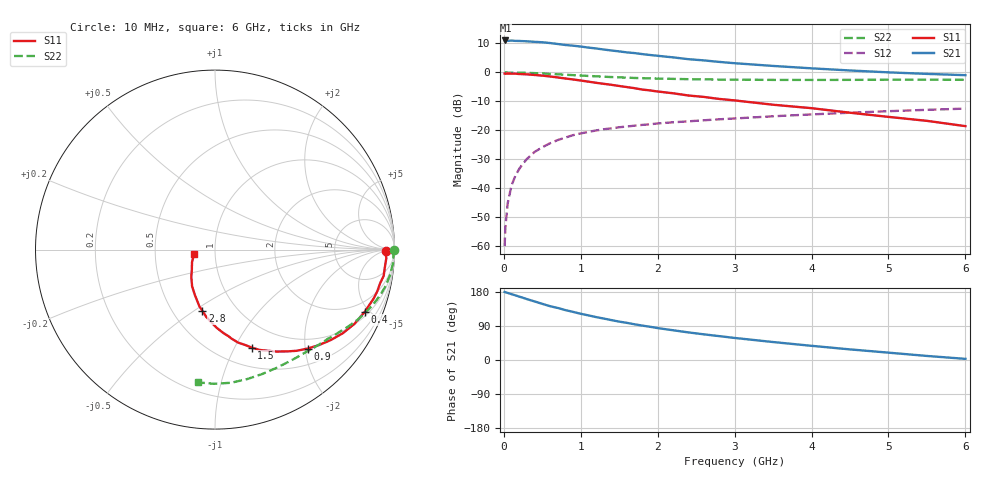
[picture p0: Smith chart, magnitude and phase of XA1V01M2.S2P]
! SIEMENS Discrete & RF Semiconductors
! BFY180
! Si NPN RF Bipolar Junction Transistor in MICRO-X
! VCE = 1 V  IC = 1.2 mA
! Common Emitter S-Parameters:  May  1997
# GHz  S  MA  R  50
!  f  S11  S21  S12  S22
! GHz  MAG  ANG  MAG  ANG  MAG  ANG  MAG  ANG
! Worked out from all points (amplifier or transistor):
!   36 points, 10 MHz to 6 GHz, reference 50 ohm
!   highest |S21| = 11.0 dB at 20 MHz (marker M1)
!   |S21| within 3 dB of that: start of sweep to 1.264 GHz
!   unconditionally stable (mu >= 1): 2.75 GHz to end of sweep
!   at 250 MHz: K = 0.10, MSG = 21.1 dB, |S12| = -31.5 dB
!   at 1.4 GHz: K = 0.65, MSG = 13.4 dB, |S12| = -19.3 dB
!   at 6 GHz: K = 1.12, MAG = 3.6 dB, |S12| = -12.5 dB
!   S11 on the Smith chart (normalised r, x): 10 MHz: 42, -8; 400 MHz: 1.24, -4.69; 900 MHz: 0.80, -2.05; 1.5 GHz: 0.71, -1.17; 2.8 GHz: 0.70, -0.54; 6 GHz: 0.79, -0.04
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0.01  0.955 -0.5  3.527 179.6  0.001 92.1  0.9953 -0.2
0.02  0.9488 -1.2  3.562 178.7  0.0021 86.0  0.9999 -0.6
0.05  0.9558 -2.8  3.506 177.0  0.0055 86.8  0.9951 -1.5
0.1  0.9515 -5.9  3.545 173.7  0.0112 86.2  0.9944 -3.1
0.2  0.9389 -11.5  3.491 167.2  0.0216 82.8  0.9895 -6.1
0.4  0.9032 -22.6  3.372 154.5  0.0424 74.8  0.9723 -12.0
0.5  0.8799 -28.1  3.316 148.2  0.051 71.0  0.9582 -14.7
0.6  0.851 -33.2  3.215 142.0  0.0597 67.9  0.9434 -17.3
0.9  0.7559 -46.8  2.894 127.0  0.0826 58.8  0.8978 -24.3
1  0.7245 -51.1  2.795 122.0  0.0885 56.5  0.884 -26.4
1.1  0.6927 -55.0  2.683 117.7  0.0939 54.3  0.8688 -28.3
1.2  0.6619 -59.1  2.589 113.2  0.0996 52.0  0.856 -30.2
1.5  0.5825 -69.5  2.305 101.3  0.113 46.9  0.821 -35.2
1.8  0.5053 -79.4  2.071 90.8  0.1242 43.2  0.7959 -39.7
2  0.4682 -84.1  1.936 84.2  0.1314 40.8  0.7833 -42.7
2.2  0.4365 -88.7  1.818 78.5  0.1377 38.5  0.7735 -45.6
2.6  0.3773 -97.5  1.612 67.7  0.1491 35.1  0.7573 -50.9
2.8  0.3484 -101.6  1.519 63.0  0.155 33.6  0.7525 -53.5
3.5  0.2767 -113.9  1.294 47.4  0.1748 28.2  0.7427 -62.6
4.5  0.2014 -131.0  1.08 28.0  0.2014 20.5  0.7433 -76.1
5.5  0.1458 -151.5  0.943 10.7  0.226 12.3  0.7477 -90.4
6  0.1181 -168.8  0.896 3.0  0.2372 7.9  0.7459 -97.5
